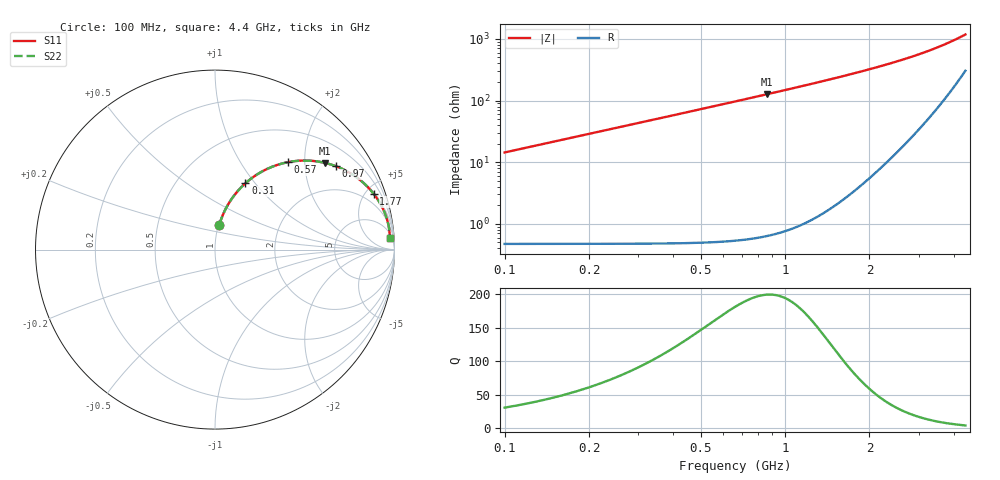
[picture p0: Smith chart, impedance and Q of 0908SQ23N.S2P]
! Coilcraft 0908SQ-23N Air Core Inductor
! 15 June 2010
# MHZ S MA R 50
!Freq  MagS11  AngS11  MagS21  AngS21  MagS12  AngS12  MagS22  AngS22
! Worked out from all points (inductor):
!   431 points, 100 MHz to 4.4 GHz, reference 50 ohm
!   read as one part in series: L = 22.9 nH near 120 MHz
!   highest Q = 200 at 860 MHz (marker M1), where L = 23.3 nH
!   S11 on the Smith chart (normalised r, x): 100 MHz: 1.01, +0.29; 310 MHz: 1.01, +0.89; 570 MHz: 1.01, +1.65; 970 MHz: 1.02, +2.87; 1.77 GHz: 1.11, +5.64; 4.4 GHz: 11, +27
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100  0.1416 80.0  0.9853 -8.2  0.9853 -8.2  0.1416 80.0
120  0.1692 78.7  0.981 -9.8  0.981 -9.8  0.1692 78.7
160  0.2231 75.9  0.9702 -12.9  0.9702 -12.9  0.2231 75.9
200  0.2751 73.0  0.9569 -16.0  0.9569 -16.0  0.2752 73.0
250  0.337 69.5  0.9371 -19.7  0.9371 -19.7  0.337 69.5
310  0.406 65.4  0.9096 -24.0  0.9096 -24.0  0.406 65.4
370  0.4688 61.5  0.8791 -28.0  0.8791 -28.0  0.4688 61.5
430  0.5254 57.8  0.8467 -31.8  0.8467 -31.8  0.5255 57.8
500  0.5839 53.8  0.8078 -35.8  0.8078 -35.8  0.5839 53.8
570  0.6348 50.1  0.7688 -39.5  0.7688 -39.5  0.6348 50.1
680  0.7012 45.0  0.7092 -44.7  0.7092 -44.7  0.7012 45.0
820  0.7661 39.5  0.6389 -50.2  0.6389 -50.2  0.7661 39.5
860  0.7814 38.2  0.6202 -51.6  0.6202 -51.6  0.7814 38.2
970  0.8173 34.7  0.572 -55.0  0.572 -55.0  0.8174 34.7
1100  0.8506 31.2  0.5211 -58.5  0.5211 -58.5  0.8507 31.2
1230  0.8764 28.2  0.4762 -61.5  0.4762 -61.5  0.8765 28.2
1540  0.9178 22.6  0.3888 -66.9  0.3888 -66.9  0.9178 22.6
1770  0.937 19.4  0.338 -69.9  0.338 -69.9  0.937 19.4
2250  0.9601 14.5  0.2576 -74.2  0.2576 -74.2  0.9601 14.5
2970  0.9741 9.5  0.1764 -77.1  0.1764 -77.1  0.9741 9.5
3690  0.9773 6.2  0.1214 -76.5  0.1214 -76.5  0.9773 6.2
4400  0.9755 3.7  0.08269 -71.4  0.08269 -71.4  0.9755 3.7
